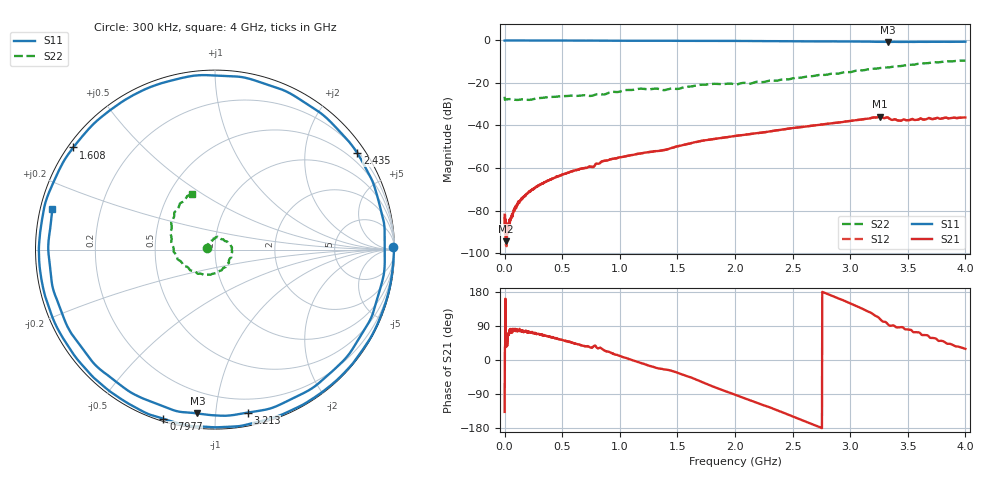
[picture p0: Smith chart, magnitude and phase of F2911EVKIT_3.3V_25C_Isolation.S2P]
! Integrated Device Technology
! Corporate Headquarters
! 6024 Silver Creek Valley Road
! San Jose, CA 95138  USA
! Phone:  1-408-284-8200
! Toll Free:  1-800-223-1366
! Webpage:  http://www.idt.com/
! Timing and RF Division
! 515 Groton Road, Suite 102
! Westford, MA 01886-6024
! Device:  F2911
! Description: 75 Ohm SPST RF Switch
! Frequency:  300 kHz to 4 GHz
! Package:  2 mm x 2 mm DFN Plastic Package: 8-pin
! Ports:  2 RF, 2 DC
!  Pin  1  = NC
!  Pin  2  = GND
!  Pin  3  = GND
!  Pin  4  = NC
!  Pin  5  = RF1	= Port 1
!  Pin  6  = VDD
!  Pin  7  = V1
!  Pin  8  = RF2	= Port 2
!  EP  = GND
! State:  Isolation
! EVKIT Voltages:		VCC	= +3.3 V
!  V1	= 0 V (Logic LOW)
! Data:  The device was measured on the F2911 EVKit
!  using a calibrated network analyzer.
!  The results below include the EVKit RF connector and
!  PCB loss effects. The reference plane is at
!  the SMA coaxial interface. Refer to the separate
!  measured thru line.s2p file for connector and PCB loss
!  and effects.
! Misc:
! Date Measured:  2017-8-11
! Date:  2017-9-21  SJ
! Note:
!  Integrated Device Technology supplies this data as a sample
!	of measured data. Data was taken at 25 degrees C.
!  Integrated Device Technology reserves the right to change
! 	this data at anytime.
!Freq	S11:SOLT2(ON)	S21:SOLT2(ON)	S12:SOLT2(ON)	S22:SOLT2(ON)
!PortZ  Port1:75+j0  Port2:75+j0
# Hz S dB R 75
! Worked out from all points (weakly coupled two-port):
!   1601 points, 300 kHz to 4 GHz, reference 75 ohm
!   highest |S21| = -35.86 dB at 3.26 GHz (marker M1); lowest = -94.4 dB at 10.3 MHz (marker M2)
!   lowest |S11| = -0.7 dB at 3.328 GHz (marker M3), VSWR 23.23, Z = 5.82 - j67.1 ohm
!   |S11| at or under -10 dB: nowhere
!   |S22| runs from -28.0 to -9.5 dB; largest |S21 - S12| = 0.00014
!   S11 on the Smith chart (normalised r, x): 300 kHz: open; 797.7 MHz: 0.01, -0.74; 1.608 GHz: 0.02, +0.32; 2.435 GHz: 0.25, +3.24; 3.213 GHz: 0.10, -1.21; 4 GHz: 0.04, +0.12
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300000  -0.09 0.7  -82.02 -137.0  -82.96 -5.1  -26.51 167.1
1.029925e7  -0.03 -1.4  -94.39 36.7  -94.01 -2.0  -27.81 179.4
7.779419e7  -0.04 -10.4  -80.86 79.9  -80.32 79.2  -27.80 175.1
3.027773e8  -0.04 -40.4  -68.02 67.6  -67.79 67.1  -27.11 150.3
4.952629e8  -0.07 -66.2  -63.29 54.1  -63.18 53.1  -26.24 137.9
6.677499e8  -0.09 -89.5  -60.29 38.5  -60.26 39.0  -25.87 124.6
7.977402e8  -0.13 -106.9  -57.90 33.2  -57.96 33.6  -25.33 110.8
1.095218e9  -0.18 -147.4  -53.96 1.1  -53.97 0.9  -23.33 85.7
1.3352e9  -0.16 -179.5  -51.96 -22.1  -52.01 -22.2  -22.81 67.7
1.607679e9  -0.24 144.2  -48.50 -45.2  -48.51 -45.1  -21.75 29.2
1.810164e9  -0.23 117.1  -46.40 -70.2  -46.44 -70.2  -20.44 7.4
2.00015e9  -0.24 92.6  -44.95 -91.9  -44.96 -91.9  -20.65 -13.8
2.207634e9  -0.30 65.0  -43.52 -115.1  -43.53 -115.2  -19.42 -43.4
2.435117e9  -0.38 34.1  -41.74 -140.6  -41.74 -140.8  -18.31 -74.3
2.6676e9  -0.48 1.8  -40.13 -168.8  -40.15 -168.9  -16.84 -104.6
2.94008e9  -0.47 -37.9  -38.32 157.5  -38.33 157.4  -15.03 -138.6
3.212559e9  -0.67 -78.7  -36.21 117.6  -36.24 117.5  -13.34 -168.8
3.260056e9  -0.65 -86.1  -35.86 108.0  -35.89 108.0  -12.96 -175.1
3.32755e9  -0.75 -96.2  -36.30 94.1  -36.32 94.0  -12.75 178.6
3.33505e9  -0.74 -97.3  -36.55 91.9  -36.57 91.9  -12.71 177.6
3.682524e9  -0.66 -149.8  -36.51 62.1  -36.52 62.0  -10.62 140.5
4e9  -0.60 166.1  -36.24 29.4  -36.26 29.3  -9.47 112.3
